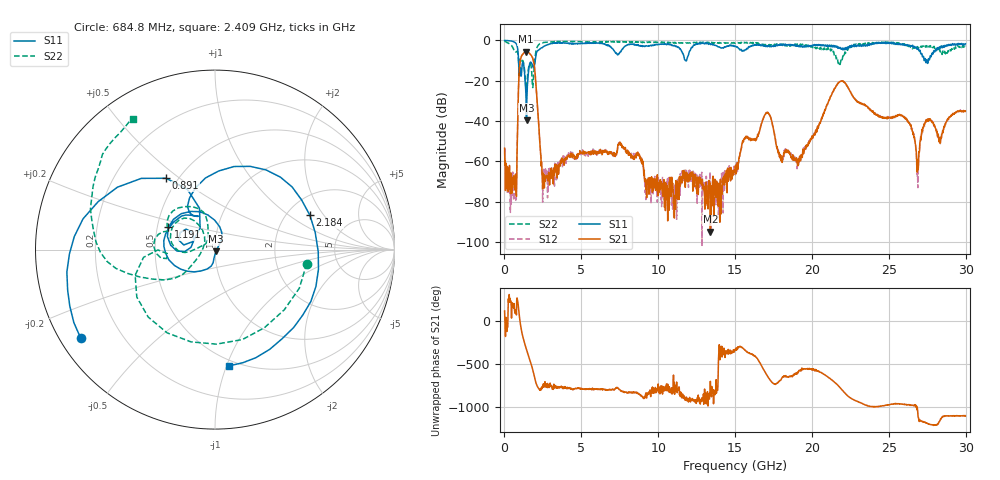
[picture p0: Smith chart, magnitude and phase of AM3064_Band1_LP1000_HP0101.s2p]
# Hz S DB R 50.0
!freq dBS11 angS11 dBS21 angS21 dBS12 angS12 dBS22 angS22
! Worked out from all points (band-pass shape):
!   1600 points, 10 MHz to 29.98 GHz, reference 50 ohm
!   highest |S21| = -5.51 dB at 1.397 GHz (marker M1); lowest = -94.8 dB at 13.39 GHz (marker M2)
!   |S21| within 3 dB of the highest: 1.075 GHz to 1.82 GHz (745.6 MHz wide, 51.5 % of centre)
!   lowest |S11| = -39.6 dB at 1.435 GHz (marker M3), VSWR 1.02, Z = 50.5 - j0.902 ohm
!   |S11| at or under -10 dB: 916.9 MHz to 1.994 GHz (1.077 GHz wide, 74 % of centre); 11.77 GHz to 11.84 GHz (66.82 MHz wide, 0.566 % of centre); 27.49016 GHz to 27.56453 GHz (74.37 MHz wide, 0.27 % of centre)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
!   |S22| runs from -24.3 to -0.3 dB; largest |S21 - S12| = 0.0065
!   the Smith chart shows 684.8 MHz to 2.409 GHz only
!   S11 on the Smith chart (normalised r, x): 684.8 MHz: 0.06, -0.30; 891 MHz: 0.43, +0.45; 1.191 GHz: 0.57, +0.15; 2.184 GHz: 2.65, +1.48; 2.409 GHz: 0.45, -1.02
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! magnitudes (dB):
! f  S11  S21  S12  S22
! 10 MHz  0.0  -53.5  -55.6  -0.3
! 684.8 MHz  -1.0  -74.1  -73.9  -5.7
! 891 MHz  -6.3  -30.1  -30.1  -7.9
! 1.191 GHz  -10.8  -6.9  -6.9  -9.9
! 1.397 GHz  -27.0  -5.5  -5.5  -24.0
! 1.435 GHz  -39.6  -5.5  -5.5  -23.6
! 1.884 GHz  -13.6  -10.0  -10.1  -18.3
! 2.184 GHz  -5.0  -36.9  -36.9  -2.5
! 2.409 GHz  -3.7  -60.1  -61.8  -1.3
! 5.015 GHz  -1.5  -55.6  -56.0  -0.6
! 7.545 GHz  -5.7  -52.1  -51.6  -0.7
! 10 GHz  -2.0  -77.0  -67.2  -0.9
! 13.39 GHz  -1.9  -94.8  -73.6  -1.2
! 15 GHz  -3.0  -65.0  -66.5  -1.4
! 17.05 GHz  -2.8  -35.9  -35.7  -2.4
! 17.99 GHz  -2.3  -59.5  -58.6  -2.3
! 19.99 GHz  -2.8  -48.4  -48.3  -3.0
! 21.9 GHz  -4.4  -20.2  -20.0  -9.4
! 25 GHz  -1.1  -38.4  -38.5  -1.1
! 26.89 GHz  -4.1  -63.1  -73.0  -3.6
! 27.49 GHz  -9.9  -39.2  -39.7  -3.1
! 29.98 GHz  -1.7  -35.1  -35.1  -3.2
